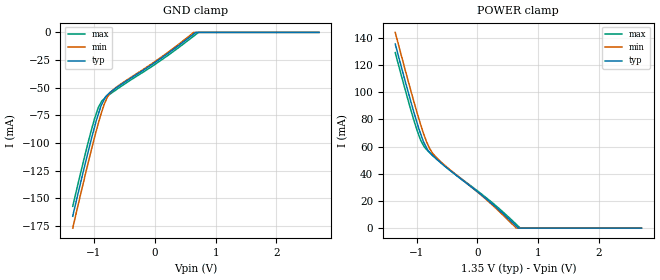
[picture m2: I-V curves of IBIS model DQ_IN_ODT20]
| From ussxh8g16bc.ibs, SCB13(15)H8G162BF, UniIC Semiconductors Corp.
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| MODEL DQ_IN_ODT20 (Data Input with 20ohm ODT, 800-2133Mbps)
[Model]   DQ_IN_ODT20
Model_type   Input
Vinl = 545.000mV
Vinh = 805.000mV
|   typ   min   max
|C_comp   1.035pF   0.986pF   1.103pF
C_comp_power_clamp   0.5175pF   0.4930pF   0.5515pF
C_comp_gnd_clamp   0.5175pF   0.4930pF   0.5515pF
| Note: C_comp changes when the ODT circuit is enabled.
[Model Spec]
| Input threshold voltage corners
Vinl   0.5450V   0.5115V   0.5825V
Vinh   0.8050V   0.7715V   0.8425V
| Dynamic Overshoot Parameters from DDR3L Specification
|D_overshoot_ampl_h   0.40   NA   NA
|D_overshoot_ampl_l   0.40   NA   NA
|D_overshoot_area_h   0.11n   NA   NA
|D_overshoot_area_l   0.11n   NA   NA
[Receiver Thresholds]
Vth   =  0.675V
Vth_min  =  0.6615V
Vth_max  =  0.6885V
Vinh_ac  =  0.130V
Vinh_dc  =  0.090V
Vinl_ac  = -0.130V
Vinl_dc  = -0.090V
Tslew_ac =  5.000ns |Not specified, so set to high value
Threshold_sensitivity = 0.50
Reference_supply Power_clamp_ref
[Voltage Range]   1.3500V   1.2830V   1.4250V
[POWER Clamp Reference]   1.3500V   1.2830V   1.4250V
| Junction Temperature (Ambient temp is 40C typ, 85C min, 0C max)
[Temperature Range]   45.0   90.0   0.0
[GND Clamp]
|   Voltage   I(typ)   I(min)   I(max)
-1.35V    -166.3mA   -177.1mA   -157.3mA
-1.11V    -110.8mA   -121mA     -102.3mA
-990mV    -85.35mA   -94.61mA   -77.81mA
-935mV    -74.97mA   -83.31mA   -68.79mA
-885mV    -66.4mA    -73.78mA   -63.4mA
-810mV    -58.2mA    -62.2mA    -58.78mA
-785mV    -56.84mA   -58.97mA   -57.76mA
-680mV    -51.97mA   -51.62mA   -53.61mA
110mV     -23.21mA   -22.26mA   -24.93mA
640mV     -1.463mA   0A         -3.331mA
718mV     0A         0A         0A
2.7V      0A         0A         0A
[POWER Clamp]
|   Voltage   I(typ)   I(min)   I(max)
-1.35V    135.5mA    144.1mA    129.2mA
-1.11V    95.68mA    103.8mA    89.59mA
-990mV    77.3mA     84.75mA    71.78mA
-930mV    69.11mA    75.86mA    64.5mA
-885mV    63.46mA    69.61mA    60.78mA
-780mV    55.58mA    58.21mA    55.37mA
-730mV    53.18mA    54.8mA     53.36mA
-590mV    47.64mA    48.4mA     47.94mA
115mV     22.74mA    22.32mA    23.5mA
640mV     1.535mA    94.48uA    2.842mA
707mV     0A         0A         0A
2.7V      0A         0A         0A
